(* Logix 5000 AddOnInstructionDefinition export AMCI_3204_AOP_Configure; software revision 20.03 *)

ADD_ON_INSTRUCTION AMCI_3204_AOP_Configure   (* revision 1.0 *)
VAR_INPUT
   channel_number : INT; {required}
   home_input : BOOL; {required}
   home_input_active_state : BOOL; {required}
   Emergency_Stop : BOOL; {required}
   Emergency_Stop_active_state : BOOL; {required}
   CW_Limit : BOOL; {required}
   CW_Limit_actitve_state : BOOL; {required}
   CCW_Limit : BOOL; {required}
   CCW_Limit_active_state : BOOL; {required}
   Backplane_Home_Proximity_Enable : BOOL;
   _0_CW_CCW_1_step_direction : BOOL; {required}
   _0_enable_1_disable_channel : BOOL;
   Starting_Speed : DINT; {required}
END_VAR
VAR_IN_OUT
   AMCi_3204_output_data : AM:1756_3204:O:0; {required}
END_VAR
VAR
   command_data_block : DINT[5];
        [0].31   // Mode Bit 1=Configuraiton Mode 0=Command Mode
END_VAR

ROUTINE Logic   (* ladder *)
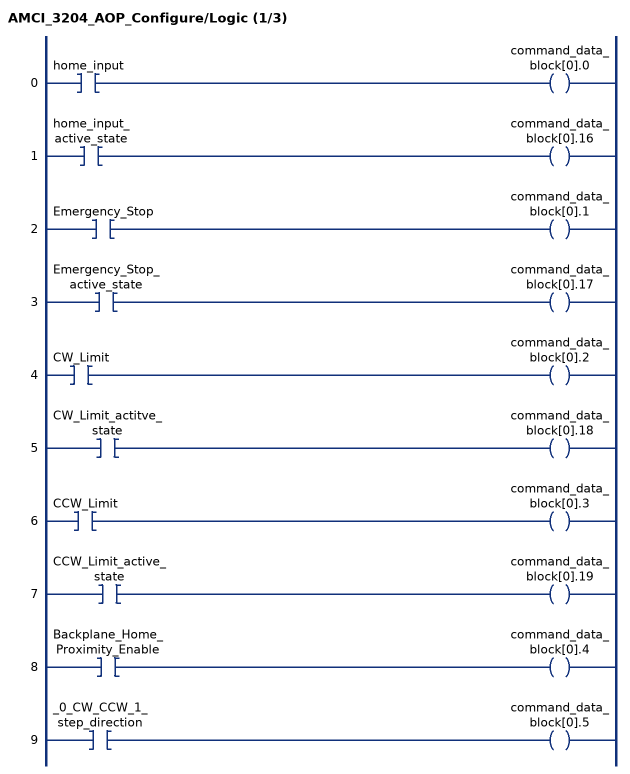
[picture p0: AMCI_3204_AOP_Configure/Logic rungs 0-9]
   0: XIC(home_input)OTE(command_data_block[0].0);
   1: XIC(home_input_active_state)OTE(command_data_block[0].16);
   2: XIC(Emergency_Stop)OTE(command_data_block[0].1);
   3: XIC(Emergency_Stop_active_state)OTE(command_data_block[0].17);
   4: XIC(CW_Limit)OTE(command_data_block[0].2);
   5: XIC(CW_Limit_actitve_state)OTE(command_data_block[0].18);
   6: XIC(CCW_Limit)OTE(command_data_block[0].3);
   7: XIC(CCW_Limit_active_state)OTE(command_data_block[0].19);
   8: XIC(Backplane_Home_Proximity_Enable)OTE(command_data_block[0].4);
   9: XIC(_0_CW_CCW_1_step_direction)OTE(command_data_block[0].5);
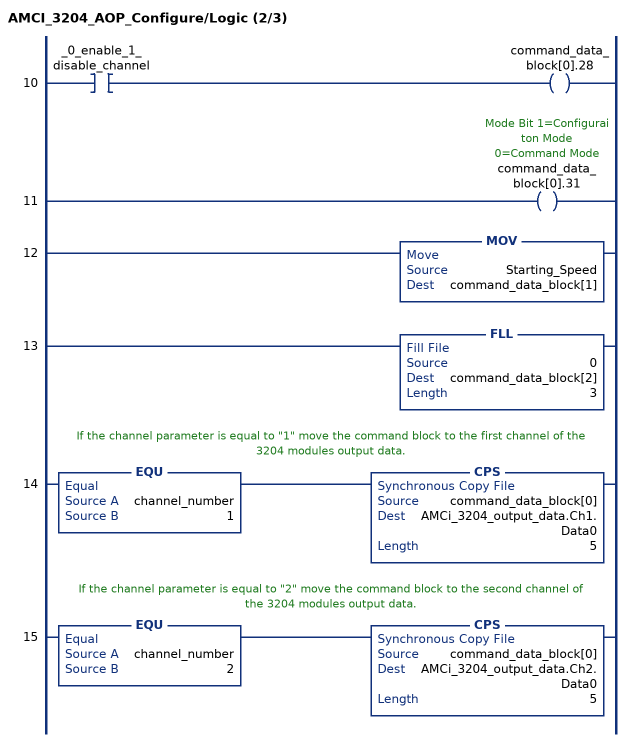
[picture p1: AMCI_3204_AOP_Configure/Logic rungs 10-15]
   10: XIC(_0_enable_1_disable_channel)OTE(command_data_block[0].28);
   11: OTE(command_data_block[0].31);
   12: MOV(Starting_Speed,command_data_block[1]);
   13: FLL(0,command_data_block[2],3);
   // If the channel parameter is equal to "1" move the command block to the first channel of the 3204 modules output data.
   14: EQU(channel_number,1)CPS(command_data_block[0],AMCi_3204_output_data.Ch1.Data0,5);
   // If the channel parameter is equal to "2" move the command block to the second channel of the 3204 modules output data.
   15: EQU(channel_number,2)CPS(command_data_block[0],AMCi_3204_output_data.Ch2.Data0,5);
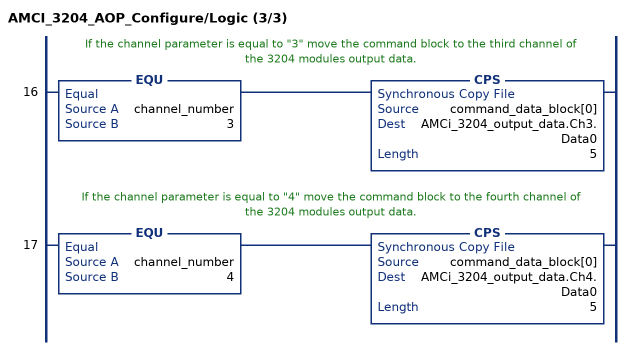
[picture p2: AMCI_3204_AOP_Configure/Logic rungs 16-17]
   // If the channel parameter is equal to "3" move the command block to the third channel of the 3204 modules output data.
   16: EQU(channel_number,3)CPS(command_data_block[0],AMCi_3204_output_data.Ch3.Data0,5);
   // If the channel parameter is equal to "4" move the command block to the fourth channel of the 3204 modules output data.
   17: EQU(channel_number,4)CPS(command_data_block[0],AMCi_3204_output_data.Ch4.Data0,5);
END_ROUTINE
END_ADD_ON_INSTRUCTION
